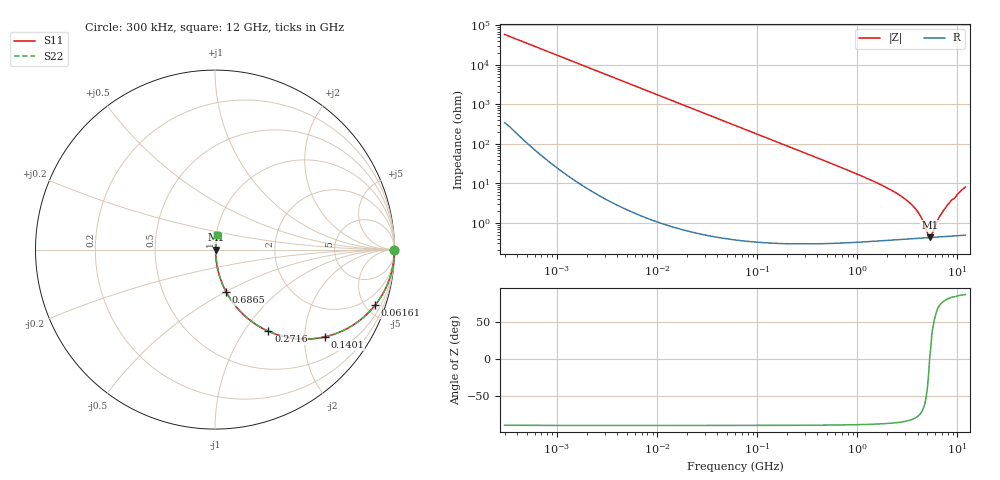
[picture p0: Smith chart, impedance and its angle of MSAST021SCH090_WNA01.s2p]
! MSAST021SCH090_WNA01  S-PARAMETER MODEL  ( General Type )
! Model Generated by TAIYO YUDEN Corporation (http://www.ty-top.com)
! Version 2.0
! TAIYO YUDEN Control No. 181101
! Copyright(c) 2015 TAIYO YUDEN CO.,LTD. All Rights Reserved.
! Product Description (link to TY-COMPAS)
! https://ds.yuden.co.jp/TYCOMPAS/or/detail?pn=MSAST021SCH090CWNA01&u=M
! Products Name : Multilayer Ceramic Capacitors
! Characteristics :
!  Capacitance : 9 pF , Rated Voltage : 25V , TCC : CH / C0H
!  Case Size : 0.25 x 0.125 / 0.0098 x 0.0049 [mm/inch] , Thickness : 0.125 / 0.0049 [mm/inch]
!  (Conditions: Temperature = 25 degC , DC Bias Current/Voltage = 0A / 0V)
! External Node Assignments :
!  1  o---| |---o  2
! GND o---------o GND
! Frequency Range : 0.3MHz  -  12000MHz  [ 401 STEP ]
# MHz S RI R 50
! Freq[MHz].  S11 Real  S11 Imag  S21 Real  S21 Imag  S12 Real  S12 Imag  S22 Real  S22 Imag
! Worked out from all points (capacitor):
!   401 points, 300 kHz to 12 GHz, reference 50 ohm
!   read as one part in series: C = 9 pF near 316.3 kHz
!   lowest |Z| = 427 mohm at 5.279 GHz (marker M1)
!   series resonance near 5.276 GHz, so ESL is about 100 pH
!   S11 on the Smith chart (normalised r, x): 300 kHz: open; 61.61 MHz: 1.01, -5.74; 140.1 MHz: 1.01, -2.52; 271.6 MHz: 1.01, -1.30; 686.5 MHz: 1.01, -0.51; 12 GHz: 1.01, +0.16
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0.3  1 -0.0017  1.28e-05 0.0017  1.28e-05 0.0017  1 -0.0017
1.769972  0.9999 -0.01  0.000109 0.01  0.000109 0.01  0.9999 -0.01
10.44266  0.9965 -0.0588  0.00351 0.0588  0.00351 0.0588  0.9965 -0.0588
26.39317  0.9781 -0.146  0.0219 0.146  0.0219 0.146  0.9781 -0.146
60  0.8964 -0.3041  0.1036 0.3041  0.1036 0.3041  0.8964 -0.3041
61.61074  0.8914 -0.3105  0.1086 0.3105  0.1086 0.3105  0.8914 -0.3105
91.67136  0.7877 -0.4081  0.2123 0.4081  0.2123 0.4081  0.7877 -0.4081
140.0606  0.6139 -0.4856  0.3861 0.4856  0.3861 0.4856  0.6139 -0.4856
271.6094  0.2974 -0.4549  0.7026 0.4549  0.7026 0.4549  0.2974 -0.4549
353.9943  0.1997 -0.3968  0.8003 0.3968  0.8003 0.3968  0.1997 -0.3968
686.4755  0.0628 -0.2366  0.9372 0.2366  0.9372 0.2366  0.0628 -0.2366
2088.533  0.00862 -0.0705  0.9914 0.0705  0.9914 0.0705  0.00862 -0.0705
2947.191  0.00551 -0.0409  0.9945 0.0409  0.9945 0.0409  0.00551 -0.0409
3740.715  0.00455 -0.0233  0.9955 0.0233  0.9955 0.0233  0.00455 -0.0233
4270.516  0.0043 -0.0142  0.9957 0.0142  0.9957 0.0142  0.0043 -0.0142
5006.236  0.00423 -0.00348  0.9958 0.00348  0.9958 0.00348  0.00423 -0.00348
5278.635  0.00425 3.86e-05  0.9957 -3.86e-05  0.9957 -3.86e-05  0.00425 3.86e-05
5565.855  0.0043 0.00304  0.9957 -0.00304  0.9957 -0.00304  0.0043 0.00304
6524.734  0.00457 0.0126  0.9954 -0.0126  0.9954 -0.0126  0.00457 0.0126
7648.807  0.0051 0.024  0.9949 -0.024  0.9949 -0.024  0.0051 0.024
10511.28  0.00823 0.0588  0.9918 -0.0588  0.9918 -0.0588  0.00823 0.0588
12000  0.0113 0.0797  0.9887 -0.0797  0.9887 -0.0797  0.0113 0.0797
